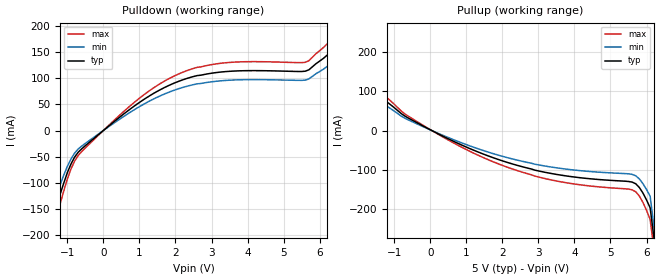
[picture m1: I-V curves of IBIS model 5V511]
[IBIS Ver]   2.1
[File name]   672_5.ibs
[File Rev]   2.0
[Date]   10/11/00
[Source]   ICS MicroClock Applications Engineering 2
[Disclaimer] This information is for modeling purposes only, and is
(C) Copyright Integrated Circuit Systems, Inc. 1997-2001
   All rights reserved
ICS hereby grants the user of this IBIS model a non-exclusive,
nontransferable license to use this IBIS model under the following terms.
Before using this IBIS model, the user should read this license.
If the user does not accept these terms,  the IBIS model should be
returned to ICS within 30 days.
   The user is granted this license only to use the IBIS model and
is not granted rights to sell, load, rent, lease or license the IBIS
model in whole or in part, or in modified form to anyone other than
user. User may modify the IBIS model to suit its specific
applications but rights to derivative works and such modifications
shall belong to ICS.
   This IBIS model is provided on an "AS IS" basis and ICS makes
absolutely no warranty with respect to the information contained
herein. ICS DISCLAIMS AND CUSTOMER WAIVES ALL WARRANTIES, EXPRESS
OR IMPLIED, INCLUDING WARRANTIES OF MERCHANTABILITY OR FITNESS FOR
A PARTICULAR PURPOSE. The entire risk as to quality and performance
is with the Customer. ACCORDINGLY, IN NO EVENT SHALL THE COMPANY BE
LIABLE FOR ANY DAMAGES, WHETHER IN CONTRACT OR TORT,INCLUDING ANY
LOST PROFITS OR OTHER INCIDENTAL, CONSEQUENTIAL, EXEMPLARY, OR
PUNITIVE DAMAGES ARISING OUT OF THE USE OR APPLICATION OF THE IBIS
model provided in this package. Further, ICS reserves the right to
make changes without notice to any product herein to improve
reliability, function, or design. ICS does not convey any license
under patent rights or any other intellectual property rights,
including those of third parties.
   ICS is not obligated to provide maintenance or support
for the licensed IBIS model.
[Component]   ICS672-01/02
[Manufacturer] Integrated Circuit Systems Inc.
[Package]
|   typ   min   max
R_pkg   40m   35m   45m
L_pkg   1.65nH   1.35nH   1.95nH
C_pkg   0.24pF   0.14pF   0.34pF
[pin]   signal_name   model_name   R_pin   L_pin   C_pin
   2   CLK90   5V511
   3   CLK180   5V511
   4   CLK270   5V511
  14   CLK0   5V511
  15   FBCLK   5V511
| Models and submodels in the file (1): 5V511 (Output)
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|   ICS672-01/02 5V Clock Drive Model
| This model is suitable for all output pins on the
| ICS672-01/02
[Model]   5V511
Model_type   Output
Polarity   Non-Inverting
|   typ   min   max
C_comp   5pF   4pF   6pF
|   typ   min   max
[Voltage range]  5.0V   4.5V   5.5V
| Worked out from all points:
|   slope of the pulldown table from 0 to 0.75 V, typ, clamps not added: 18.2 ohm
|   slope of the pullup table from 0 to 0.75 V, typ, clamps not added: 22.3 ohm
[pulldown]
|Voltage I (typ)   I (min)   I (max)
-5V       -3A        -3A        -3A
-1.5V     -193.1mA   -164.1mA   -222.1mA
-1.4V     -168.4mA   -143.1mA   -193.6mA
-1V       -80.51mA   -68.43mA   -92.59mA
-700mV    -41.56mA   -35.32mA   -47.79mA
1V        53.72mA    45.66mA    61.78mA
2.3V      99.18mA    84.31mA    114.1mA
3.5V      113.2mA    96.22mA    130.2mA
5.6V      113.4mA    96.41mA    130.4mA
6.3V      150.5mA    128mA      173.1mA
6.6V      197.9mA    168.2mA    227.6mA
10V       3A         3A         3A
[pullup]
|Voltage I (typ)   I (min)   I (max)
-5V       3A         3A         3A
-2.4V     200.1mA    170.1mA    230.1mA
-2.1V     144mA      122.4mA    165.6mA
-2V       133.7mA    113.7mA    153.8mA
-800mV    42.62mA    36.23mA    49.01mA
600mV     -25.37mA   -21.56mA   -29.17mA
1.9V      -73.85mA   -62.77mA   -84.93mA
3.5V      -111.3mA   -94.59mA   -128mA
5.6V      -130.8mA   -111.2mA   -150.4mA
5.8V      -144.5mA   -122.8mA   -166.1mA
6.1V      -196.1mA   -166.7mA   -225.6mA
10V       -3A        -3A        -3A
[Ramp]
|   typ   min   max
dV/dt_r   2.07/0.39n   1.97/0.43n   2.17/0.35n
dV/dt_f   2.21/0.43n   2.10/0.47n   2.32/0.39n
